| IBIS file p1022_ibis_feb24.ibs generated by Viper version: 2010.02.15
[IBIS Ver]   3.2
[Comment Char]   |_char
[File Name]   p1022_ibis_mar2.ibs
[File Rev]   rev1.0
[Date]   Thu Feb 25 16:07:44 2010
[Source]   Generated using: Viper
[Notes]   updated RLC data
[Disclaimer] IMPORTANT NOTICE
  This information is provided on an AS IS basis and without warranty.
  IN NO EVENT SHALL Freescale BE LIABLE FOR INCIDENTAL OR CONSEQUENTIAL
  DAMAGES ARISING FROM USE OF THIS INFORMATION. THIS DISCLAIMER OF
  WARRANTY EXTENDS TO THE USER OF THE INFORMATION, AND TO THEIR CUSTOMERS
  OR USERS OF PRODUCTS  AND IS IN LIEU OF ALL WARRANTIES WHETHER EXPRESS,
  IMPLIED, OR STATUTORY, INCLUDING IMPLIED WARRANTIES OF MERCHANTABILITY
  OR FITNESS FOR PARTICULAR PURPOSE.
  Freescale does not represent or warrant that the information furnished
  hereunder is free of infringement of any third party patents,
  copyrights, trade secrets, or other intellectual property rights.
  Freescale does not represent or warrant that the information is free of
  defect, or that it meets any particular standard, requirements or need
  of the user of the infomation or their customers.
  Freescale reserves the right to change the information in this file
  without notice.
[Copyright]   (C) Copyright Freescale 2004 - 2010, All Rights Reserved.
|   P1022
[Component]   P1022
[Manufacturer]   FREESCALE
[Package]
| variable   typ   min   max
R_pkg   0.7016960   0.214305   0.869311
L_pkg   7.73384nH   3.69979nH   11.5388nH
C_pkg   1.99730pF   1.32765pF   2.81449pF
[Pin] signal_name   model_name   R_pin   L_pin   C_pin
A1   VSS   GND   NA   NA   NA
A2   VSS   GND   NA   NA   NA
A3   MDQ39   ddr   0.747982  9.70333nH 2.59253pF
A4   GVDD   POWER   NA   NA   NA
A5   MDM05   ddr   0.717482  9.33185nH 1.99975pF
A6   VSS   GND   NA   NA   NA
A7   MDQ47   ddr   0.729467  9.16668nH 2.03973pF
A8   GVDD   POWER   NA   NA   NA
A9   MDQ54   ddr   0.735149  8.13776nH 1.76304pF
A10   GVDD   POWER   NA   NA   NA
A11   MDM07   ddr   0.694958  8.68017nH 1.68609pF
A12   VSS   GND   NA   NA   NA
A13   MDQ63   ddr   0.685751  8.11112nH 1.93324pF
A14   VSS   GND   NA   NA   NA
A15   LAD10   lvcmos   0.777971  8.37697nH 1.67142pF
A16   LAD04   lvcmos   0.700731  8.2178nH  1.9126pF
A17   LAD01   lvcmos   0.75683   8.57406nH 1.87132pF
A18   LAD26   lvcmos   0.760623  8.65983nH 1.85274pF
A19   LAD23   lvcmos   0.766493  8.93644nH 1.743pF
A20   LAD20   lvcmos   0.766971  8.96903nH 1.89829pF
A21   LAD17   lvcmos   0.702347  8.7987nH  1.5871pF
A22   LCS0_B   lvcmos   0.722144  8.74151nH 2.06773pF
A23   VSS   GND   NA   NA   NA
A24   LCLK0   lvcmos   0.808004  9.97666nH 2.20396pF
A25   LCLK1   lvcmos   0.748103  9.5762nH  2.27038pF
A26   VSS   GND   NA   NA   NA
A27   TEMP_CATHODE   POWER   0.751033  9.87414nH 2.26105pF
A28   VSS   GND   NA   NA   NA
A29   VSS   GND   NA   NA   NA
B1   GVDD   POWER   NA   NA   NA
B2   MDQ38   ddr   0.809458  9.97646nH 2.37608pF
B3   VSS   GND   NA   NA   NA
B4   MDQ35   ddr   0.675651  9.29962nH 2.53862pF
B5   MDQ41   ddr   0.754296  9.20264nH 1.96462pF
B6   MDQS05   ddr   0.748763  9.62507nH 2.47055pF
B7   MDQ46   ddr   0.762222  8.92197nH 2.02782pF
B8   MDQ43   ddr   0.708598  8.50501nH 2.08974pF
B9   VSS   GND   NA   NA   NA
B10   MDQ56   ddr   0.741395  8.31025nH 1.94339pF
B11   MDQ57   ddr   0.739117  8.28462nH 1.86747pF
B12   MDQS07   ddr   0.684389  8.73644nH 2.31pF
B13   MDQ62   ddr   0.727662  7.77585nH 1.85543pF
B14   MDQ59   ddr   0.732429  8.00584nH 1.99911pF
B15   LAD11   lvcmos   0.692875  7.49306nH 1.85047pF
B16   LAD05   lvcmos   0.740501  7.94284nH 1.94522pF
B17   LAD02   lvcmos   0.657515  7.76898nH 1.91602pF
B18   VSS   GND   NA   NA   NA
B19   LAD24   lvcmos   0.745003  8.28546nH 1.80061pF
B20   BVDD   POWER   NA   NA   NA
B21   LAD16   lvcmos   0.75217   8.53668nH 1.54649pF
B22   VSS   GND   NA   NA   NA
B23   LWE1_B   lvcmos   0.768453  8.82719nH 1.99814pF
B24   LGPL3   lvcmos   0.720038  8.68977nH 2.09379pF
B25   BVDD   POWER   NA   NA   NA
B26   TEMP_ANODE   POWER   0.800236  9.45775nH 2.23395pF
B27   SPI_CS0_B   lvcmos   0.77681   9.69603nH 2.32325pF
B28   SPI_CS1_B   lvcmos   0.6984   9.31032nH 2.73683pF
B29   VSS   GND   NA   NA   NA
C1   MDQS_B04   ddr   0.792078  9.83271nH 2.57031pF
C2   MDQS04   ddr   0.705702  9.28383nH 2.67801pF
C3   MDM04   ddr   0.71794   9.26539nH 2.42861pF
C4   MDQ34   ddr   0.656881  8.4244nH  2.48774pF
C5   MDQ40   ddr   0.707344  8.62866nH 2.31281pF
C6   MDQS_B05   ddr   0.674196  9.08304nH 2.48388pF
C7   GVDD   POWER   NA   NA   NA
C8   MDQ42   ddr   0.728676  7.7836nH  2.00625pF
C9   MDQS06   ddr   0.653727  7.64321nH 2.03409pF
C10   MDQ60   ddr   0.674331  7.73856nH 2.07298pF
C11   MDQ61   ddr   0.654937  7.13965nH 1.98477pF
C12   MDQS_B07   ddr   0.750121  9.30784nH 2.09011pF
C13   VSS   GND   NA   NA   NA
C14   MDQ58   ddr   0.663714  7.96634nH 1.72058pF
C15   BVDD   POWER   NA   NA   NA
C16   LAD06   lvcmos   0.656701  7.05135nH 1.93021pF
C17   LAD03   lvcmos   0.719406  7.36586nH 1.95061pF
C18   LDP1   lvcmos   0.724029  7.50077nH 1.87876pF
C19   LAD22   lvcmos   0.661298  7.35622nH 1.83935pF
C20   LAD19   lvcmos   0.730113  7.78479nH 1.7538pF
C21   LCS2_B   lvcmos   0.739806  7.92256nH 1.93931pF
C22   LGPL0   lvcmos   0.745588  8.03202nH 2.076pF
C23   LALE   lvcmos   0.750517  8.2294nH  2.09312pF
C24   LGPL4   lvcmos   0.765139  8.58843nH 2.06771pF
C25   SPI_MOSI   lvcmos   0.705009  8.35195nH 2.26877pF
C26   VSS   GND   NA   NA   NA
C27   SPI_CS2_B   lvcmos   0.734144  9.07613nH 2.2447pF
C28   SDHC_DAT1   lvcmos   0.696295  9.23289nH 2.50112pF
C29   SDHC_CLK   lvcmos   0.831498  10.5218nH 2.28529pF
D1   GVDD   POWER   NA   NA   NA
D2   MDQ37   ddr   0.76027   9.50741nH 2.12906pF
D3   MDQ33   ddr   0.807158  9.50311nH 2.13208pF
D4   MDQ44   ddr   0.627315  7.98496nH 2.36865pF
D5   VSS   GND   NA   NA   NA
D6   MDQ45   ddr   0.620035  7.41491nH 2.27755pF
D7   MDQ48   ddr   0.712654  7.33209nH 2.20401pF
D8   MDQ49   ddr   0.71175   7.38798nH 1.96456pF
D9   MDQS_B06   ddr   0.719441  7.97825nH 2.07488pF
D10   GVDD   POWER   NA   NA   NA
D11   MDQ51   ddr   0.731452  7.99976nH 1.93683pF
D12   GVDD   POWER   NA   NA   NA
D13   LAD14   lvcmos   0.687323  6.47207nH 1.51203pF
D14   LAD13   lvcmos   0.643595  6.56045nH 1.6414pF
D15   LAD12   lvcmos   0.710721  6.70823nH 1.78542pF
D16   LAD07   lvcmos   0.69999   6.92713nH 1.83412pF
D17   VSS   GND   NA   NA   NA
D18   LAD27   lvcmos   0.644075  6.59265nH 1.76486pF
D19   BVDD   POWER   NA   NA   NA
D20   LAD18   lvcmos   0.71132   7.2312nH  1.79978pF
D21   VSS   GND   NA   NA   NA
D22   LBCTL   lvcmos   0.662836  6.99163nH 2.16362pF
D23   BVDD   POWER   NA   NA   NA
D24   LGPL5   lvcmos   0.685726  7.65156nH 2.17734pF
D25   SPI_CLK   lvcmos   0.667534  7.73941nH 2.15435pF
D26   SDHC_DAT0   lvcmos   0.722686  8.33496nH 2.81449pF
D27   SDHC_DAT2   lvcmos   0.769674  9.19593nH 2.36132pF
D28   UART_SIN0   lvcmos   0.818963  9.51209nH 2.34724pF
D29   VSS   GND   NA   NA   NA
E1   MODT01   ddr   0.768945  9.58951nH 2.06186pF
E2   MODT03   ddr   0.745012  9.04779nH 2.23177pF
E3   VSS   GND   NA   NA   NA
E4   MDQ36   ddr   0.71465   8.3374nH  2.12026pF
E5   MDQ32   ddr   0.723452  8.04595nH 2.22862pF
E6   GVDD   POWER   NA   NA   NA
E7   MDQ52   ddr   0.651886  7.21957nH 1.96438pF
E8   GVDD   POWER   NA   NA   NA
E9   VSS   GND   NA   NA   NA
E10   MDQ55   ddr   0.694918  6.93545nH 1.8336pF
E11   VSS   GND   NA   NA   NA
E12   MDIC00   ddr   0.671948  5.99856nH 1.66456pF
E13   LAD15   lvcmos   0.631894  6.71174nH 1.63833pF
E14   VSS   GND   NA   NA   NA
E15   BVDD   POWER   NA   NA   NA
E16   LAD09   lvcmos   0.619147  5.85899nH 1.8411pF
E17   LAD08   lvcmos   0.623017  5.91538nH 1.856pF
E18   LAD00   lvcmos   0.622408  6.07334nH 1.7523pF
E19   LAD21   lvcmos   0.626555  6.12834nH 1.9256pF
E20   LCS1_B   lvcmos   0.635442  6.17821nH 1.82914pF
E21   LWE0_B   lvcmos   0.638292  6.39312nH 2.00511pF
E22   LGPL2   lvcmos   0.711723  7.01223nH 2.1374pF
E23   DIU_DE   lvcmos   0.718933  7.195nH   2.22906pF
E24   VSS   GND   NA   NA   NA
E25   SPI_CS3_B   lvcmos   0.593703  6.90482nH 2.23741pF
E26   SDHC_DAT3   lvcmos   0.663694  7.64798nH 2.35593pF
E27   OVDD   POWER   NA   NA   NA
E28   UART_SIN1   lvcmos   0.814474  9.39955nH 2.28045pF
E29   SSI_TXD   lvcmos   0.773615  9.5324nH  2.30058pF
F1   MODT00   ddr   0.767477  9.43676nH 2.13559pF
F2   MODT02   ddr   0.81492   9.35608nH 2.1323pF
F3   MA13   ddr   0.784095  8.73301nH 2.18083pF
F4   VSS   GND   NA   NA   NA
F5   MCS_B01   ddr   0.749609  7.70032nH 2.17327pF
F6   MCS_B03   ddr   0.73552   7.35365nH 2.19972pF
F7   VSS   GND   NA   NA   NA
F8   MDQ53   ddr   0.643059  6.74904nH 2.00573pF
F9   GVDD   POWER   NA   NA   NA
F10   MDM06   ddr   0.636797  6.68012nH 2.05382pF
F11   MDQ50   ddr   0.632859  6.51846nH 2.07728pF
F12   MDIC01   ddr   0.593766  6.03687nH 1.60187pF
F13   VSS   GND   NA   NA   NA
F14   SENSEVDD   POWER   0.628311  5.49999nH 1.65526pF
F15   SENSEVSS   GND   NA   NA   NA
F16   BVDD   POWER   NA   NA   NA
F17   LDP0   lvcmos   0.607637  5.50127nH 1.79259pF
F18   LAD25   lvcmos   0.594032  5.39975nH 1.72445pF
F19   LCS3_B   lvcmos   0.62234   5.84429nH 1.83376pF
F20   BVDD   POWER   NA   NA   NA
F21   LGPL1   lvcmos   0.62597   5.69382nH 1.58857pF
F22   BVDD   POWER   NA   NA   NA
F23   SPI_MISO   lvcmos   0.694828  6.68908nH 1.77993pF
F24   SDHC_CMD   lvcmos   0.581608  6.4253nH  2.77594pF
F25   SDHC_WP   lvcmos   0.736041  7.52883nH 2.1004pF
F26   SSI_TFS   lvcmos   0.776554  8.45125nH 1.93089pF
F27   UART_RTS0_B   lvcmos   0.791654  8.73106nH 2.23647pF
F28   UART_SOUT0   lvcmos   0.735462  8.53016nH 2.17307pF
F29   OVDD   POWER   NA   NA   NA
G1   MWE_B   ddr   0.81798   9.63755nH 2.09559pF
G2   MCS_B00   ddr   0.73876   8.49107nH 2.12548pF
G3   GVDD   POWER   NA   NA   NA
G4   MCS_B02   ddr   0.675974  7.31698nH 2.09895pF
G5   VSS   GND   NA   NA   NA
G6   MCAS_B   ddr   0.670224  6.89342nH 2.23097pF
G9   AVDD_CORE0   POWER   0.310257  5.00716nH 2.08432pF
G10   VSS   GND   NA   NA   NA
G20   AVDD_CORE1   POWER   0.235846  3.9426nH  1.77074pF
G21   VSS   GND   NA   NA   NA
G24   SDHC_CD   lvcmos   0.615851  5.79493nH 1.8637pF
G25   OVDD   POWER   NA   NA   NA
G26   SSI_TCK   lvcmos   0.67726   7.08006nH 1.88322pF
G27   VSS   GND   NA   NA   NA
G28   IIC1_SCL   lvcmos   0.731176  8.33606nH 1.99554pF
G29   CKSTP_IN1_B   lvcmos   0.810997  9.63909nH 1.96353pF
H1   VSS   GND   NA   NA   NA
H2   MCK_B00   ddr   0.68165   7.52908nH 2.11178pF
H3   MCK00   ddr   0.750375  8.08883nH 2.14795pF
H4   VSS   GND   NA   NA   NA
H5   MBA00   ddr   0.742889  7.21161nH 1.88577pF
H6   MRAS_B   ddr   0.652761  6.3406nH  2.02834pF
H24   UART_SOUT1   lvcmos   0.650936  6.02915nH 2.17556pF
H25   CKSTP_IN0_B   lvcmos   0.67136   6.76601nH 2.04482pF
H26   UART_RTS1_B   lvcmos   0.756241  7.7748nH  1.95949pF
H27   CKSTP_OUT0_B   lvcmos   0.706241  8.02652nH 2.07119pF
H28   UDE1_B   lvcmos   0.712269  8.21792nH 2.17731pF
H29   VSS   GND   NA   NA   NA
J1   MA00   ddr   0.796246  9.22816nH 1.84503pF
J2   VSS   GND   NA   NA   NA
J3   GVDD   POWER   NA   NA   NA
J4   MA10   ddr   0.686989  7.12046nH 1.84029pF
J5   MBA01   ddr   0.734781  6.97896nH 1.77277pF
J6   GVDD   POWER   NA   NA   NA
J7   MVREF   POWER   0.267911  3.89422nH 2.45211pF
J23   UART_CTS1_B   lvcmos   0.629162  5.35462nH 2.03577pF
J24   IIC1_SDA   lvcmos   0.639074  5.71514nH 1.9761pF
J25   OVDD   POWER   NA   NA   NA
J26   IRQ10   lvcmos   0.67645   7.06237nH 2.08085pF
J27   IRQ11   lvcmos   0.754726  8.10729nH 2.08486pF
J28   IRQ_OUT_B   lvcmos   0.758499  8.45336nH 1.95538pF
J29   SRESET_B   lvcmos   0.869311  11.5388nH 2.11591pF
K1   GVDD   POWER   NA   NA   NA
K2   MCK02   ddr   0.665769  7.15095nH 2.13736pF
K3   MCK_B02   ddr   0.726796  7.62398nH 2.00158pF
K4   GVDD   POWER   NA   NA   NA
K5   MA01   ddr   0.708382  6.56449nH 1.78235pF
K6   VSS   GND   NA   NA   NA
K7   VSS   GND   NA   NA   NA
K10   VDD   POWER   NA   NA   NA
K11   VDD   POWER   NA   NA   NA
K12   VDD   POWER   NA   NA   NA
K13   VDD   POWER   NA   NA   NA
K14   VDD   POWER   NA   NA   NA
K15   VDD   POWER   NA   NA   NA
K16   VDD   POWER   NA   NA   NA
K17   VDD   POWER   NA   NA   NA
K18   VDD   POWER   NA   NA   NA
K19   VDD   POWER   NA   NA   NA
K20   VDD   POWER   NA   NA   NA
K23   VSS   GND   NA   NA   NA
K24   UART_CTS0_B   lvcmos   0.693565  5.94257nH 1.83568pF
K25   MCP1_B   lvcmos   0.699642  6.50366nH 2.07126pF
K26   MCP0_B   lvcmos   0.66247   6.85144nH 2.1763pF
K27   IRQ06   lvcmos   0.681091  7.56841nH 2.1623pF
K28   IRQ08   lvcmos   0.76863   8.68056nH 2.1677pF
K29   OVDD   POWER   NA   NA   NA
L1   MCK_B03   ddr   0.734922  8.03983nH 2.05312pF
L2   MCK03   ddr   0.67263   7.55603nH 2.02095pF
L3   VSS   GND   NA   NA   NA
L4   MA03   ddr   0.727973  7.28074nH 1.7884pF
L5   GVDD   POWER   NA   NA   NA
L6   MA02   ddr   0.629357  5.53765nH 1.6768pF
L10   VDD   POWER   NA   NA   NA
L11   VSS   GND   NA   NA   NA
L12   VSS   GND   NA   NA   NA
L13   VSS   GND   NA   NA   NA
L14   VSS   GND   NA   NA   NA
L15   VSS   GND   NA   NA   NA
L16   VSS   GND   NA   NA   NA
L17   VSS   GND   NA   NA   NA
L18   VSS   GND   NA   NA   NA
L19   VSS   GND   NA   NA   NA
L20   VDD   POWER   NA   NA   NA
L24   CKSTP_OUT1_B   lvcmos   0.689227  6.02751nH 1.83644pF
L25   TRIG_IN   lvcmos   0.69154   6.35757nH 1.71564pF
L26   VSS   GND   NA   NA   NA
L27   READY_P1   lvcmos   0.727793  7.67494nH 1.94516pF
L28   IRQ09   lvcmos   0.669829  7.35824nH 2.016pF
L29   TRST_B   lvcmos   0.75249   8.62062nH 1.87616pF
M1   VSS   GND   NA   NA   NA
M2   MA06   ddr   0.747102  7.96217nH 2.03621pF
M3   MA08   ddr   0.668586  6.99082nH 1.96255pF
M4   VSS   GND   NA   NA   NA
M5   MA05   ddr   0.676039  5.77571nH 1.60285pF
M6   MA04   ddr   0.616647  5.3732nH  1.62193pF
M10   VDD   POWER   NA   NA   NA
M11   VSS   GND   NA   NA   NA
M12   VSS   GND   NA   NA   NA
M13   VSS   GND   NA   NA   NA
M14   VSS   GND   NA   NA   NA
M15   VSS   GND   NA   NA   NA
M16   VSS   GND   NA   NA   NA
M17   VSS   GND   NA   NA   NA
M18   VSS   GND   NA   NA   NA
M19   VSS   GND   NA   NA   NA
M20   VDD   POWER   NA   NA   NA
M24   UDE0_B   lvcmos   0.604684  5.30535nH 1.82263pF
M25   TRIG_OUT   lvcmos   0.605211  5.52842nH 1.69668pF
M26   TMS   lvcmos   0.680323  6.47272nH 1.71661pF
M27   TEST_SEL_B   lvcmos   0.641802  6.5438nH  2.01703pF
M28   TDO   lvcmos   0.661586  7.48518nH 1.77687pF
M29   CLK_OUT   lvcmos   0.74508   9.50959nH 2.26363pF
N1   MA07   ddr   0.760278  8.53997nH 1.82525pF
N2   GVDD   POWER   NA   NA   NA
N3   MCK04   ddr   0.62391   6.12413nH 1.8762pF
N4   MCK_B04   ddr   0.689124  6.60337nH 1.94903pF
N5   MA11   ddr   0.629666  5.97326nH 1.7484pF
N6   GVDD   POWER   NA   NA   NA
N10   VDD   POWER   NA   NA   NA
N11   VSS   GND   NA   NA   NA
N12   VSS   GND   NA   NA   NA
N13   VSS   GND   NA   NA   NA
N14   VSS   GND   NA   NA   NA
N15   VSS   GND   NA   NA   NA
N16   VSS   GND   NA   NA   NA
N17   VSS   GND   NA   NA   NA
N18   VSS   GND   NA   NA   NA
N19   VSS   GND   NA   NA   NA
N20   VDD   POWER   NA   NA   NA
N24   O2VDD   POWER   NA   NA   NA
N25   IRQ07   lvcmos   0.706639  7.122nH   1.78275pF
N26   TCK   lvcmos   0.632794  6.45982nH 1.6978pF
N27   OVDD   POWER   NA   NA   NA
N28   TDI   lvcmos   0.669808  7.83522nH 1.92322pF
N29   VSS   GND   NA   NA   NA
P1   MA09   ddr   0.761782  8.66565nH 1.91017pF
P2   MA12   ddr   0.734634  7.84455nH 1.77566pF
P3   GVDD   POWER   NA   NA   NA
P4   MA14   ddr   0.640481  6.35886nH 1.88735pF
P5   VSS   GND   NA   NA   NA
P6   MA15   ddr   0.600726  5.18608nH 1.6909pF
P10   VDDC   POWER   NA   NA   NA
P11   VSS   GND   NA   NA   NA
P12   VSS   GND   NA   NA   NA
P13   VSS   GND   NA   NA   NA
P14   VSS   GND   NA   NA   NA
P15   VSS   GND   NA   NA   NA
P16   VSS   GND   NA   NA   NA
P17   VSS   GND   NA   NA   NA
P18   VSS   GND   NA   NA   NA
P19   VSS   GND   NA   NA   NA
P20   VDD   POWER   NA   NA   NA
P24   AVDD_PLAT   POWER   0.225725  3.91717nH 1.70343pF
P25   BVDD_VSEL1   lvcmos   0.583695  5.28241nH 1.66388pF
P26   SCAN_MODE_B   lvcmos   0.723151  7.58863nH 2.37353pF
P27   HRESET_B   lvcmos   0.626681  6.547nH   1.76201pF
P28   HRESET_REQ_B   lvcmos   0.724556  7.83466nH 1.78084pF
P29   SYS_CLK_IN   lvcmos   0.744299  8.45424nH 1.65183pF
R1   MECC03   ddr   0.696247  8.27557nH 1.97882pF
R2   MECC07   ddr   0.73996   8.13322nH 1.94202pF
R3   MCK01   ddr   0.621499  6.22548nH 1.78015pF
R4   MCK_B01   ddr   0.686242  6.72345nH 1.84929pF
R5   GVDD   POWER   NA   NA   NA
R6   MBA02   ddr   0.587662  4.86479nH 1.66315pF
R10   VDDC   POWER   NA   NA   NA
R11   VSS   GND   NA   NA   NA
R12   VSS   GND   NA   NA   NA
R13   VSS   GND   NA   NA   NA
R14   VSS   GND   NA   NA   NA
R15   VSS   GND   NA   NA   NA
R16   VSS   GND   NA   NA   NA
R17   VSS   GND   NA   NA   NA
R18   VSS   GND   NA   NA   NA
R19   VSS   GND   NA   NA   NA
R20   VDD   POWER   NA   NA   NA
R24   POWER_OK   lvcmos   0.586072  5.21871nH 1.74996pF
R25   VSS   GND   NA   NA   NA
R26   BVDD_VSEL0   lvcmos   0.668531  6.22835nH 1.78343pF
R27   LVDD_VSEL   lvcmos   0.639598  6.84039nH 1.83973pF
R28   SENSEVDDC   POWER   0.667936  7.68638nH 1.76873pF
R29   O2VDD   POWER   NA   NA   NA
T1   MECC02   ddr   0.74095   8.15796nH 1.92604pF
T2   MECC06   ddr   0.67143   7.48077nH 1.88371pF
T3   VSS   GND   NA   NA   NA
T4   MCK05   ddr   0.671192  6.22963nH 1.85988pF
T5   MCK_B05   ddr   0.604507  5.63884nH 1.97876pF
T6   VSS   GND   NA   NA   NA
T10   VDD   POWER   NA   NA   NA
T11   VSS   GND   NA   NA   NA
T12   VSS   GND   NA   NA   NA
T13   VSS   GND   NA   NA   NA
T14   VSS   GND   NA   NA   NA
T15   VSS   GND   NA   NA   NA
T16   VSS   GND   NA   NA   NA
T17   VSS   GND   NA   NA   NA
T18   VSS   GND   NA   NA   NA
T19   VSS   GND   NA   NA   NA
T20   VDD1C   POWER   NA   NA   NA
T24   IRQ05   lvcmos   0.589086  5.2944nH  1.95022pF
T25   ASLEEP   lvcmos   0.667301  6.10241nH 1.63205pF
T26   IRQ00   lvcmos   0.687158  6.76086nH 1.74101pF
T27   O2VDD   POWER   NA   NA   NA
T28   IRQ04   lvcmos   0.726744  8.01525nH 1.73347pF
T29   RTC_CLK   lvcmos   0.69783   8.57303nH 1.96035pF
U1   VSS   GND   NA   NA   NA
U2   MDQS08   ddr   0.716988  7.89065nH 1.98034pF
U3   MDQS_B08   ddr   0.652329  7.35067nH 2.09729pF
U4   MCKE01   ddr   0.705471  6.98965nH 1.98496pF
U5   GVDD   POWER   NA   NA   NA
U6   MCKE00   ddr   0.592512  5.08767nH 1.81435pF
U10   VDD   POWER   NA   NA   NA
U11   VSS   GND   NA   NA   NA
U12   VSS   GND   NA   NA   NA
U13   VSS   GND   NA   NA   NA
U14   VSS   GND   NA   NA   NA
U15   VSS   GND   NA   NA   NA
U16   VSS   GND   NA   NA   NA
U17   VSS   GND   NA   NA   NA
U18   VSS   GND   NA   NA   NA
U19   VSS   GND   NA   NA   NA
U20   VDD1C   POWER   NA   NA   NA
U24   IRQ03   lvcmos   0.601269  5.57921nH 1.84659pF
U25   VSS   GND   NA   NA   NA
U26   USB1_NXT   lvcmos   0.629338  6.45057nH 1.69032pF
U27   POWER_EN   lvcmos   0.644821  7.00555nH 1.74565pF
U28   IRQ01   lvcmos   0.729463  8.04877nH 1.86148pF
U29   IRQ02   lvcmos   0.752273  8.79128nH 1.80881pF
V1   MDM08   ddr   0.746958  8.29642nH 1.83805pF
V2   MECC01   ddr   0.668827  7.31868nH 1.90491pF
V3   VSS   GND   NA   NA   NA
V4   MCKE02   ddr   0.711189  7.17234nH 1.94967pF
V5   VSS   GND   NA   NA   NA
V6   MCKE03   ddr   0.605909  5.48656nH 1.80924pF
V10   VDD   POWER   NA   NA   NA
V11   VSS   GND   NA   NA   NA
V12   VSS   GND   NA   NA   NA
V13   VSS   GND   NA   NA   NA
V14   VSS   GND   NA   NA   NA
V15   VSS   GND   NA   NA   NA
V16   VSS   GND   NA   NA   NA
V17   VSS   GND   NA   NA   NA
V18   VSS   GND   NA   NA   NA
V19   VSS   GND   NA   NA   NA
V20   VDD   POWER   NA   NA   NA
V24   USB1_D3   lvcmos   0.607322  5.71096nH 1.75879pF
V25   USB1_D1   lvcmos   0.65881   5.76643nH 1.66699pF
V26   USB1_D0   lvcmos   0.618288  6.01963nH 1.89407pF
V27   L2VDD   POWER   NA   NA   NA
V28   USB1_DIR   lvcmos   0.715894  7.56709nH 1.98495pF
V29   USB1_STP   lvcmos   0.752319  8.69895nH 1.6905pF
W1   GVDD   POWER   NA   NA   NA
W2   MECC05   ddr   0.731698  7.85348nH 1.90405pF
W3   MECC00   ddr   0.65613   6.92897nH 1.99099pF
W4   VSS   GND   NA   NA   NA
W5   MDQ27   ddr   0.702912  6.60364nH 1.93405pF
W6   VSS   GND   NA   NA   NA
W10   VDD   POWER   NA   NA   NA
W11   VSS   GND   NA   NA   NA
W12   VSS   GND   NA   NA   NA
W16   VSS   GND   NA   NA   NA
W18   VSS   GND   NA   NA   NA
W19   VSS   GND   NA   NA   NA
W20   VDD   POWER   NA   NA   NA
W24   USB1_D5   lvcmos   0.620582  6.10759nH 1.88772pF
W25   VSS   GND   NA   NA   NA
W26   USB1_D4   lvcmos   0.711238  7.34956nH 1.81292pF
W27   USB1_CLK   lvcmos   0.673707  7.77621nH 1.87247pF
W28   USB1_D2   lvcmos   0.74607   8.38541nH 1.79201pF
W29   VSS   GND   NA   NA   NA
Y1   MECC04   ddr   0.744797  8.23151nH 1.9271pF
Y2   MDQ19   ddr   0.703654  8.40512nH 2.13386pF
Y3   VSS   GND   NA   NA   NA
Y4   MDQ26   ddr   0.645595  6.29946nH 1.83215pF
Y5   MDQ31   ddr   0.716708  6.94691nH 1.80488pF
Y6   GVDD   POWER   NA   NA   NA
Y7   GVDD   POWER   NA   NA   NA
Y10   AVDD_DDR   POWER   0.214305  3.69979nH 1.95615pF
Y11   VDD   POWER   NA   NA   NA
Y12   VDD   POWER   NA   NA   NA
Y16   VDD   POWER   NA   NA   NA
Y18   VDD   POWER   NA   NA   NA
Y19   VDD   POWER   NA   NA   NA
Y20   VDD   POWER   NA   NA   NA
Y23   VSS   GND   NA   NA   NA
Y24   USB1_D7   lvcmos   0.617006  6.02818nH 1.96398pF
Y25   USB1_D6   lvcmos   0.697804  6.9541nH  1.80869pF
Y26   TSEC1_RXD2   lvcmos   0.715351  7.38259nH 1.75853pF
Y27   L2VDD   POWER   NA   NA   NA
Y28   TSEC1_RXD1   lvcmos   0.688816  7.99755nH 1.91339pF
Y29   TSEC1_GTX_CLK125   lvcmos   0.771088  9.03453nH 1.87871pF
AA1   MDQ18   ddr   0.795809  9.69339nH 2.17107pF
AA2   MDQ23   ddr   0.709076  8.49571nH 2.17933pF
AA3   MDQ22   ddr   0.771421  8.9429nH  2.1567pF
AA4   GVDD   POWER   NA   NA   NA
AA5   MDQ30   ddr   0.6549   6.57618nH 1.87999pF
AA6   MDM03   ddr   0.66511   6.7596nH  2.0776pF
AA7   VSS   GND   NA   NA   NA
AA23  TSEC1_RXD3   lvcmos   0.689364  6.28487nH 1.98785pF
AA24  TSEC1_RX_DV   lvcmos   0.722191  7.43464nH 1.96713pF
AA25  L2VDD   POWER   NA   NA   NA
AA26  TSEC1_RXD0   lvcmos   0.662609  7.05028nH 1.86096pF
AA27  TSEC1_TXD3   lvcmos   0.752433  8.17827nH 2.01611pF
AA28  TSEC1_TX_EN   lvcmos   0.719164  8.93363nH 2.05205pF
AA29  VSS   GND   NA   NA   NA
AB1   VSS   GND   NA   NA   NA
AB2   MDQS02   ddr   0.751456  8.86427nH 2.41421pF
AB3   MDQS_B02   ddr   0.687495  8.3718nH  2.47445pF
AB4   MDQS_B03   ddr   0.646093  6.5114nH  2.21966pF
AB5   MDQS03   ddr   0.708597  7.03821nH 2.25397pF
AB6   GVDD   POWER   NA   NA   NA
AB24  TSEC2_RX_CLK   lvcmos   0.69745   6.16275nH 1.7061pF
AB25  TSEC1_TXD2   lvcmos   0.730216  7.19852nH 2.02132pF
AB26  VSS   GND   NA   NA   NA
AB27  TSEC1_TXD0   lvcmos   0.763196  8.31969nH 1.92929pF
AB28  TSEC1_TXD1   lvcmos   0.710356  8.2521nH  2.02809pF
AB29  TSEC1_RX_CLK   lvcmos   0.724709  8.99529nH 1.95072pF
AC1   MDM02   ddr   0.720921  8.90853nH 2.00523pF
AC2   MDQ17   ddr   0.791928  9.39064nH 2.15356pF
AC3   MDQ21   ddr   0.777352  8.80939nH 2.26867pF
AC4   VSS   GND   NA   NA   NA
AC5   MDQ25   ddr   0.738948  7.43405nH 1.92245pF
AC6   MDQ29   ddr   0.736137  7.39419nH 2.18276pF
AC20  SD_IMP_CAL_TX2   tx_pzctl   0.698084  5.35753nH 1.85591pF
AC21  X2VSS   GND   NA   NA   NA
AC24  TSEC2_TXD0   lvcmos   0.62913   6.59453nH 2.02328pF
AC25  LVDD   POWER   NA   NA   NA
AC26  TSEC2_GTX_CLK   lvcmos   0.756982  7.92708nH 2.05207pF
AC27  TSEC2_RXD3   lvcmos   0.75544   8.04661nH 2.17475pF
AC28  TSEC2_RX_DV   lvcmos   0.709701  8.08989nH 2.19683pF
AC29  VSS   GND   NA   NA   NA
AD1   MDQ16   ddr   0.747121  9.47092nH 2.23892pF
AD2   MDQ20   ddr   0.73457   8.97058nH 2.35503pF
AD3   GVDD   POWER   NA   NA   NA
AD4   MDQ28   ddr   0.757823  8.00645nH 1.98016pF
AD5   MDQ24   ddr   0.691876  7.46687nH 2.01299pF
AD6   VSS   GND   NA   NA   NA
AD7   DDRCLK   lvcmos   0.725731  7.80904nH 1.81614pF
AD8   XVSS   GND   NA   NA   NA
AD9   SD_TXA_P   lynx_tx   0.767153  7.41281nH 1.57434pF
AD10  XVDD   POWER   NA   NA   NA
AD11  SDAVDD   POWER   0.665957  7.35563nH 1.39528pF
AD12  SDAVSS   GND   NA   NA   NA
AD13  SD_PLL_TPA   opdalg_out   0.661314  6.02375nH 1.54654pF
AD14  XVDD   POWER   NA   NA   NA
AD15  SD_TXF_P   lynx_tx   0.723625  6.18732nH 1.32765pF
AD16  XVSS   GND   NA   NA   NA
AD17  X2VSS   GND   NA   NA   NA
AD18  SD_PLL_TPD2   pouv_out   0.672646  5.57979nH 1.66844pF
AD19  SDAVDD2   POWER   0.638341  6.25359nH 1.59881pF
AD20  X2VSS   GND   NA   NA   NA
AD21  SD_TXE_N2   lynx_tx   0.734851  6.65032nH 1.7116pF
AD22  X2VDD   POWER   NA   NA   NA
AD23  VSS   GND   NA   NA   NA
AD24  TSEC_1588_CLK_OUT   lvcmos   0.66378   6.98275nH 2.72173pF
AD25  TSEC2_TXD1   lvcmos   0.746153  8.30497nH 2.80784pF
AD26  FA_VDD   POWER   0.761131  8.05443nH 2.19663pF
AD27  TSEC2_RXD2   lvcmos   0.715598  8.22195nH 2.13812pF
AD28  POVDD   POWER   0.730029  8.63467nH 1.9705pF
AD29  TSEC1_GTX_CLK   lvcmos   0.749816  9.2186nH  2.21955pF
AE1   VSS   GND   NA   NA   NA
AE2   MDQ11   ddr   0.752689  9.44986nH 2.10991pF
AE3   MDQ10   ddr   0.79641   9.30975nH 2.071pF
AE4   VSS   GND   NA   NA   NA
AE5   MDQ15   ddr   0.622086  7.14341nH 2.26945pF
AE6   MDQ14   ddr   0.675537  9.03836nH 2.40484pF
AE7   VSS   GND   NA   NA   NA
AE8   XVDD   POWER   NA   NA   NA
AE9   SD_TXA_N   lynx_tx   0.776672  7.05759nH 1.73301pF
AE10  SD_TXB_P   lynx_tx   0.694223  7.03079nH 1.77516pF
AE11  XVSS   GND   NA   NA   NA
AE12  SD_PLL_TPD   pouv_out   0.743327  6.15765nH 1.67568pF
AE13  XVSS   GND   NA   NA   NA
AE14  SD_TXE_P   lynx_tx   0.663139  7.05245nH 1.6831pF
AE15  SD_TXF_N   lynx_tx   0.727544  6.01318nH 1.49367pF
AE16  XVDD   POWER   NA   NA   NA
AE17  SD_TXA_P2   lynx_tx   0.736953  6.83502nH 1.44397pF
AE18  X2VDD   POWER   NA   NA   NA
AE19  SDAVSS2   GND   NA   NA   NA
AE20  X2VSS   GND   NA   NA   NA
AE21  SD_TXE_P2   lynx_tx   0.735237  6.65822nH 1.74802pF
AE22  X2VDD   POWER   NA   NA   NA
AE23  VSS   GND   NA   NA   NA
AE24  TSEC_1588_PULSE_OUT1 lvcmos   0.583265  6.98743nH 2.71577pF
AE25  LVDD   POWER   NA   NA   NA
AE26  TSEC2_TX_EN   lvcmos   0.781846  8.8613nH  2.0133pF
AE27  VSS   GND   NA   NA   NA
AE28  TSEC2_RXD1   lvcmos   0.816418  9.65856nH 2.25875pF
AE29  LVDD   POWER   NA   NA   NA
AF1   MDQS01   ddr   0.74139   10.8726nH 2.72838pF
AF2   GVDD   POWER   NA   NA   NA
AF3   MDM01   ddr   0.791041  9.38409nH 2.37806pF
AF4   MDQ08   ddr   0.740629  8.79748nH 2.27745pF
AF5   MDQ12   ddr   0.716996  8.35449nH 2.38214pF
AF6   GVDD   POWER   NA   NA   NA
AF7   VSS   GND   NA   NA   NA
AF8   XVSS   GND   NA   NA   NA
AF9   XVSS   GND   NA   NA   NA
AF10  SD_TXB_N   lynx_tx   0.698896  6.93622nH 1.80151pF
AF11  XVDD   POWER   NA   NA   NA
AF12  SD_REF_CLK_B   ptrmr100_cm   0.704775  7.61118nH 1.70107pF
AF13  XVDD   POWER   NA   NA   NA
AF14  SD_TXE_N   lynx_tx   0.659113  6.50531nH 1.65965pF
AF15  XVSS   GND   NA   NA   NA
AF16  SD_IMP_CAL_TX   tx_pzctl   0.726209  6.62944nH 1.79653pF
AF17  SD_TXA_N2   lynx_tx   0.735773  6.79387nH 1.50033pF
AF18  S2VSS   GND   NA   NA   NA
AF19  SD_PLL_TPA2   opdalg_out   0.7577   6.94577nH 1.82348pF
AF20  X2VDD   POWER   NA   NA   NA
AF21  S2VSS   GND   NA   NA   NA
AF22  X2VSS   GND   NA   NA   NA
AF24  VSS   GND   NA   NA   NA
AF25  VSS   GND   NA   NA   NA
AF26  TSEC_1588_ALARM_OUT1 lvcmos   0.640101  8.1342nH  2.27843pF
AF27  TSEC2_TXD3   lvcmos   0.717311  8.94031nH 2.29889pF
AF28  VSS   GND   NA   NA   NA
AF29  TSEC2_RXD0   lvcmos   0.777582  9.96458nH 2.2087pF
AG1   MDQS_B01   ddr   0.811159  11.4708nH 2.54042pF
AG2   MDQ09   ddr   0.751936  9.77961nH 2.19936pF
AG3   MDQ03   ddr   0.679181  8.92513nH 2.58718pF
AG4   VSS   GND   NA   NA   NA
AG5   MDQS00   ddr   0.703516  9.84203nH 2.74267pF
AG6   MDQ01   ddr   0.687546  8.33583nH 2.25869pF
AG7   VSS   GND   NA   NA   NA
AG8   SD_IMP_CAL_RX   rx_pzctl   0.802968  8.32078nH 1.97143pF
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[Pin Mapping]   pulldown_ref   pullup_ref
A1   VSS   NC
A2   VSS   NC
A3   NC   GVDD
A4   NC   GVDD
A5   NC   GVDD
A6   VSS   NC
A7   NC   GVDD
A8   NC   GVDD
A9   NC   GVDD
A10   NC   GVDD
A11   NC   GVDD
A12   VSS   NC
A13   NC   GVDD
A14   VSS   NC
A15   NC   BVDD
A16   NC   BVDD
A17   NC   BVDD
A18   NC   BVDD
A19   NC   BVDD
A20   NC   BVDD
A21   NC   BVDD
A22   NC   BVDD
A23   VSS   NC
A24   NC   BVDD
A25   NC   BVDD
A26   VSS   NC
A27   NC   BVDD
A28   VSS   NC
A29   VSS   NC
B1   NC   GVDD
B2   NC   GVDD
B3   VSS   NC
B4   NC   GVDD
B5   NC   GVDD
B6   NC   GVDD
B7   NC   GVDD
B8   NC   GVDD
B9   VSS   NC
B10   NC   GVDD
B11   NC   GVDD
B12   NC   GVDD
B13   NC   GVDD
B14   NC   GVDD
B15   NC   BVDD
B16   NC   BVDD
B17   NC   BVDD
B18   VSS   NC
B19   NC   BVDD
B20   NC   BVDD
B21   NC   BVDD
B22   VSS   NC
B23   NC   BVDD
B24   NC   BVDD
B25   NC   BVDD
B26   NC   BVDD
B27   NC   BVDD
B28   NC   BVDD
B29   VSS   NC
C1   NC   GVDD
C2   NC   GVDD
C3   NC   GVDD
C4   NC   GVDD
C5   NC   GVDD
C6   NC   GVDD
C7   NC   GVDD
C8   NC   GVDD
C9   NC   GVDD
C10   NC   GVDD
C11   NC   GVDD
C12   NC   GVDD
C13   VSS   NC
C14   NC   GVDD
C15   NC   BVDD
C16   NC   BVDD
C17   NC   BVDD
C18   NC   BVDD
C19   NC   BVDD
C20   NC   BVDD
C21   NC   BVDD
C22   NC   BVDD
C23   NC   BVDD
C24   NC   BVDD
C25   NC   BVDD
C26   VSS   NC
C27   NC   BVDD
C28   NC   OVDD
C29   NC   OVDD
D1   NC   GVDD
D2   NC   GVDD
D3   NC   GVDD
D4   NC   GVDD
D5   VSS   NC
D6   NC   GVDD
D7   NC   GVDD
D8   NC   GVDD
D9   NC   GVDD
D10   NC   GVDD
D11   NC   GVDD
D12   NC   GVDD
D13   NC   BVDD
D14   NC   BVDD
D15   NC   BVDD
D16   NC   BVDD
D17   VSS   NC
D18   NC   BVDD
D19   NC   BVDD
D20   NC   BVDD
D21   VSS   NC
D22   NC   BVDD
D23   NC   BVDD
D24   NC   BVDD
D25   NC   BVDD
D26   NC   OVDD
D27   NC   OVDD
D28   NC   OVDD
D29   VSS   NC
E1   NC   GVDD
E2   NC   GVDD
E3   VSS   NC
E4   NC   GVDD
E5   NC   GVDD
E6   NC   GVDD
E7   NC   GVDD
E8   NC   GVDD
E9   VSS   NC
E10   NC   GVDD
E11   VSS   NC
E12   NC   GVDD
E13   NC   BVDD
E14   VSS   NC
E15   NC   BVDD
E16   NC   BVDD
E17   NC   BVDD
E18   NC   BVDD
E19   NC   BVDD
E20   NC   BVDD
E21   NC   BVDD
E22   NC   BVDD
E23   NC   BVDD
E24   VSS   NC
E25   NC   BVDD
E26   NC   OVDD
E27   NC   OVDD
E28   NC   OVDD
E29   NC   OVDD
F1   NC   GVDD
F2   NC   GVDD
F3   NC   GVDD
F4   VSS   NC
F5   NC   GVDD
F6   NC   GVDD
F7   VSS   NC
F8   NC   GVDD
F9   NC   GVDD
F10   NC   GVDD
F11   NC   GVDD
F12   NC   GVDD
F13   VSS   NC
F14   NC   BVDD
F15   SENSEVSS   NC
F16   NC   BVDD
F17   NC   BVDD
F18   NC   BVDD
F19   NC   BVDD
F20   NC   BVDD
F21   NC   BVDD
F22   NC   BVDD
F23   NC   BVDD
F24   NC   OVDD
F25   NC   OVDD
F26   NC   OVDD
F27   NC   OVDD
F28   NC   OVDD
F29   NC   OVDD
G1   NC   GVDD
G2   NC   GVDD
G3   NC   GVDD
G4   NC   GVDD
G5   VSS   NC
G6   NC   GVDD
G9   NC   AVDD_CORE0
G10   VSS   NC
G20   NC   AVDD_CORE1
G21   VSS   NC
G24   NC   OVDD
G25   NC   OVDD
G26   NC   OVDD
G27   VSS   NC
G28   NC   OVDD
G29   NC   OVDD
H1   VSS   NC
H2   NC   GVDD
H3   NC   GVDD
H4   VSS   NC
H5   NC   GVDD
H6   NC   GVDD
H24   NC   OVDD
H25   NC   OVDD
H26   NC   OVDD
H27   NC   OVDD
H28   NC   OVDD
H29   VSS   NC
J1   NC   GVDD
J2   VSS   NC
J3   NC   GVDD
J4   NC   GVDD
J5   NC   GVDD
J6   NC   GVDD
J7   NC   GVDD
J23   NC   OVDD
J24   NC   OVDD
J25   NC   OVDD
J26   NC   OVDD
J27   NC   OVDD
J28   NC   OVDD
J29   NC   OVDD
K1   NC   GVDD
K2   NC   GVDD
K3   NC   GVDD
K4   NC   GVDD
K5   NC   GVDD
K6   VSS   NC
K7   VSS   NC
K10   NC   VDD
K11   NC   VDD
K12   NC   VDD
K13   NC   VDD
K14   NC   VDD
K15   NC   VDD
K16   NC   VDD
K17   NC   VDD
K18   NC   VDD
K19   NC   VDD
K20   NC   VDD
K23   VSS   NC
K24   NC   OVDD
K25   NC   OVDD
K26   NC   OVDD
K27   NC   OVDD
K28   NC   OVDD
K29   NC   OVDD
L1   NC   GVDD
L2   NC   GVDD
L3   VSS   NC
L4   NC   GVDD
L5   NC   GVDD
L6   NC   GVDD
L10   NC   VDD
L11   VSS   NC
L12   VSS   NC
L13   VSS   NC
L14   VSS   NC
L15   VSS   NC
L16   VSS   NC
L17   VSS   NC
L18   VSS   NC
L19   VSS   NC
L20   NC   VDD
L24   NC   OVDD
L25   NC   OVDD
L26   VSS   NC
L27   NC   O2VDD
L28   NC   OVDD
L29   NC   O2VDD
M1   VSS   NC
M2   NC   GVDD
M3   NC   GVDD
M4   VSS   NC
M5   NC   GVDD
M6   NC   GVDD
M10   NC   VDD
M11   VSS   NC
M12   VSS   NC
M13   VSS   NC
M14   VSS   NC
M15   VSS   NC
M16   VSS   NC
M17   VSS   NC
M18   VSS   NC
M19   VSS   NC
M20   NC   VDD
M24   NC   OVDD
M25   NC   O2VDD
M26   NC   O2VDD
M27   NC   O2VDD
M28   NC   O2VDD
M29   NC   OVDD
N1   NC   GVDD
N2   NC   GVDD
N3   NC   GVDD
N4   NC   GVDD
N5   NC   GVDD
N6   NC   GVDD
N10   NC   VDD
N11   VSS   NC
N12   VSS   NC
N13   VSS   NC
N14   VSS   NC
N15   VSS   NC
N16   VSS   NC
N17   VSS   NC
N18   VSS   NC
N19   VSS   NC
N20   NC   VDD
N24   NC   O2VDD
N25   NC   OVDD
N26   NC   O2VDD
N27   NC   OVDD
N28   NC   O2VDD
N29   VSS   NC
P1   NC   GVDD
P2   NC   GVDD
P3   NC   GVDD
P4   NC   GVDD
P5   VSS   NC
P6   NC   GVDD
P10   NC   VDDC
P11   VSS   NC
P12   VSS   NC
P13   VSS   NC
P14   VSS   NC
P15   VSS   NC
P16   VSS   NC
P17   VSS   NC
P18   VSS   NC
P19   VSS   NC
P20   NC   VDD
P24   NC   O2VDD
P25   NC   O2VDD
P26   NC   O2VDD
P27   NC   O2VDD
P28   NC   O2VDD
P29   NC   O2VDD
R1   NC   GVDD
R2   NC   GVDD
R3   NC   GVDD
R4   NC   GVDD
R5   NC   GVDD
R6   NC   GVDD
R10   NC   VDDC
R11   VSS   NC
R12   VSS   NC
R13   VSS   NC
R14   VSS   NC
R15   VSS   NC
R16   VSS   NC
R17   VSS   NC
R18   VSS   NC
R19   VSS   NC
R20   NC   VDD
R24   NC   O2VDD
R25   VSS   NC
R26   NC   O2VDD
R27   NC   O2VDD
R28   NC   O2VDD
R29   NC   O2VDD
T1   NC   GVDD
T2   NC   GVDD
T3   VSS   NC
T4   NC   GVDD
T5   NC   GVDD
T6   VSS   NC
T10   NC   VDD
T11   VSS   NC
T12   VSS   NC
T13   VSS   NC
T14   VSS   NC
T15   VSS   NC
T16   VSS   NC
T17   VSS   NC
T18   VSS   NC
T19   VSS   NC
T20   NC   VDD1C
T24   NC   O2VDD
T25   NC   O2VDD
T26   NC   O2VDD
T27   NC   O2VDD
T28   NC   O2VDD
T29   NC   O2VDD
U1   VSS   NC
U2   NC   GVDD
U3   NC   GVDD
U4   NC   GVDD
U5   NC   GVDD
U6   NC   GVDD
U10   NC   VDD
U11   VSS   NC
U12   VSS   NC
U13   VSS   NC
U14   VSS   NC
U15   VSS   NC
U16   VSS   NC
U17   VSS   NC
U18   VSS   NC
U19   VSS   NC
U20   NC   VDD1C
U24   NC   O2VDD
U25   VSS   NC
U26   NC   L2VDD
U27   NC   O2VDD
U28   NC   O2VDD
U29   NC   O2VDD
V1   NC   GVDD
V2   NC   GVDD
V3   VSS   NC
V4   NC   GVDD
V5   VSS   NC
V6   NC   GVDD
V10   NC   VDD
V11   VSS   NC
V12   VSS   NC
V13   VSS   NC
V14   VSS   NC
V15   VSS   NC
V16   VSS   NC
V17   VSS   NC
V18   VSS   NC
V19   VSS   NC
V20   NC   VDD
V24   NC   L2VDD
V25   NC   L2VDD
V26   NC   L2VDD
V27   NC   L2VDD
V28   NC   L2VDD
V29   NC   L2VDD
W1   NC   GVDD
W2   NC   GVDD
W3   NC   GVDD
W4   VSS   NC
W5   NC   GVDD
W6   VSS   NC
W10   NC   VDD
W11   VSS   NC
W12   VSS   NC
W16   VSS   NC
W18   VSS   NC
W19   VSS   NC
W20   NC   VDD
W24   NC   L2VDD
W25   VSS   NC
W26   NC   L2VDD
W27   NC   L2VDD
W28   NC   L2VDD
W29   VSS   NC
Y1   NC   GVDD
Y2   NC   GVDD
Y3   VSS   NC
Y4   NC   GVDD
Y5   NC   GVDD
Y6   NC   GVDD
Y7   NC   GVDD
Y10   NC   AVDD_DDR
Y11   NC   VDD
Y12   NC   VDD
Y16   NC   VDD
Y18   NC   VDD
Y19   NC   VDD
Y20   NC   VDD
Y23   VSS   NC
Y24   NC   L2VDD
Y25   NC   L2VDD
Y26   NC   L2VDD
Y27   NC   L2VDD
Y28   NC   L2VDD
Y29   NC   L2VDD
AA1   NC   GVDD
AA2   NC   GVDD
AA3   NC   GVDD
AA4   NC   GVDD
AA5   NC   GVDD
AA6   NC   GVDD
AA7   VSS   NC
AA23   NC   L2VDD
AA24   NC   L2VDD
AA25   NC   L2VDD
AA26   NC   L2VDD
AA27   NC   L2VDD
AA28   NC   L2VDD
AA29   VSS   NC
AB1   VSS   NC
AB2   NC   GVDD
AB3   NC   GVDD
AB4   NC   GVDD
AB5   NC   GVDD
AB6   NC   GVDD
AB24   NC   LVDD
AB25   NC   L2VDD
AB26   VSS   NC
AB27   NC   L2VDD
AB28   NC   L2VDD
AB29   NC   L2VDD
AC1   NC   GVDD
AC2   NC   GVDD
AC3   NC   GVDD
AC4   VSS   NC
AC5   NC   GVDD
AC6   NC   GVDD
AC20   NC   NC
AC21   X2VSS   NC
AC24   NC   LVDD
AC25   NC   LVDD
AC26   NC   LVDD
AC27   NC   LVDD
AC28   NC   LVDD
AC29   VSS   NC
AD1   NC   GVDD
AD2   NC   GVDD
AD3   NC   GVDD
AD4   NC   GVDD
AD5   NC   GVDD
AD6   VSS   NC
AD7   NC   O2VDD
AD8   XVSS   NC
AD9   NC   NC
AD10   NC   XVDD
AD11   NC   SDAVDD
AD12   SDAVSS   NC
AD13   NC   NC
AD14   NC   XVDD
AD15   NC   NC
AD16   XVSS   NC
AD17   X2VSS   NC
AD18   NC   NC
AD19   NC   SDAVDD2
AD20   X2VSS   NC
AD21   NC   NC
AD22   NC   X2VDD
AD23   VSS   NC
AD24   NC   LVDD
AD25   NC   LVDD
AD26   NC   LVDD
AD27   NC   LVDD
AD28   NC   LVDD
AD29   NC   L2VDD
AE1   VSS   NC
AE2   NC   GVDD
AE3   NC   GVDD
AE4   VSS   NC
AE5   NC   GVDD
AE6   NC   GVDD
AE7   VSS   NC
AE8   NC   XVDD
AE9   NC   NC
AE10   NC   NC
AE11   XVSS   NC
AE12   NC   NC
AE13   XVSS   NC
AE14   NC   NC
AE15   NC   NC
AE16   NC   XVDD
AE17   NC   NC
AE18   NC   X2VDD
AE19   SDAVSS2   NC
AE20   X2VSS   NC
AE21   NC   NC
AE22   NC   X2VDD
AE23   VSS   NC
AE24   NC   LVDD
AE25   NC   LVDD
AE26   NC   LVDD
AE27   VSS   NC
AE28   NC   LVDD
AE29   NC   LVDD
AF1   NC   GVDD
AF2   NC   GVDD
AF3   NC   GVDD
AF4   NC   GVDD
AF5   NC   GVDD
AF6   NC   GVDD
AF7   VSS   NC
AF8   XVSS   NC
AF9   XVSS   NC
AF10   NC   NC
AF11   NC   XVDD
AF12   NC   NC
AF13   NC   XVDD
AF14   NC   NC
AF15   XVSS   NC
AF16   NC   NC
AF17   NC   NC
AF18   S2VSS   NC
AF19   NC   NC
AF20   NC   X2VDD
AF21   S2VSS   NC
AF22   X2VSS   NC
AF24   VSS   NC
AF25   VSS   NC
AF26   NC   LVDD
AF27   NC   LVDD
AF28   VSS   NC
AF29   NC   LVDD
AG1   NC   GVDD
AG2   NC   GVDD
AG3   NC   GVDD
AG4   VSS   NC
AG5   NC   GVDD
AG6   NC   GVDD
AG7   VSS   NC
AG8   NC   NC
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| Diff Pairs
[Diff pin]   inv_pin   vdiff   tdelay_typ   tdelay_min   tdelay_max
|   MCK Signals
   H3   H2   250mV   0ns   NA   NA
   R3   R4   250mV   0ns   NA   NA
   K2   K3   250mV   0ns   NA   NA
   L2   L1   250mV   0ns   NA   NA
   N3   N4   250mV   0ns   NA   NA
   T4   T5   250mV   0ns   NA   NA
|   MDQS Signals: Use this format to arrange MDQS signals for
|   differential operation.  To use MDQS as
|   single-ended operation, comment out the following
|   nine lines.
   AG5   AH5   250mV   0ns   NA   NA
   AF1   AG1   250mV   0ns   NA   NA
   AB2   AB3   250mV   0ns   NA   NA
   AB5   AB4   250mV   0ns   NA   NA
   C2   C1   250mV   0ns   NA   NA
   B6   C6   250mV   0ns   NA   NA
   C9   D9   250mV   0ns   NA   NA
   B12   C12   250mV   0ns   NA   NA
   U2   U3   250mV   0ns   NA   NA
|   LYNX16 differential ports
|   SD_TX(0:3)
   AD9   AE9   NA   NA   NA   NA
   AE10   AF10   NA   NA   NA   NA
   AE14   AF14   NA   NA   NA   NA
   AD15   AE15   NA   NA   NA   NA
|   SD_RX(0:3)
   AH9   AJ9   NA   NA   NA   NA
   AH11   AJ11   NA   NA   NA   NA
   AH13   AJ13   NA   NA   NA   NA
   AH15   AJ15   NA   NA   NA   NA
|   SD_REF_CLK
   AG12   AF12   NA   NA   NA   NA
| LYNX18 differential ports
|   SD_TX(0:1)
   AE17   AF17   NA   NA   NA   NA
   AE21   AD21   NA   NA   NA   NA
|   SD_RX(0:1)
   AG18   AH18   NA   NA   NA   NA
   AH21   AG21   NA   NA   NA   NA
|   SD_REF_CLK
   AJ20   AJ19   NA   NA   NA   NA
|*   Model Selector   *
[Model Selector] ddr
ddr2_rcvr_150   DDR2 receiver with odt = 150 ohms
ddr2_rcvr_50   DDR2 receiver with odt =  50 ohms
ddr2_rcvr_75   DDR2 receiver with odt =  75 ohms
ddr2_rcvr_noterm   DDR2 receiver with no odt
ddr3_rcvr_120   DDR3 receiver with odt = 120 ohms
ddr3_rcvr_60   DDR3 receiver with odt = 60 ohms
ddr3_rcvr_noterm   DDR3 receiver with no odt
ddr2_drvr_18   DDR2 driver - 18 Ohm
ddr2_drvr_35   DDR2 driver - 35 Ohm
ddr3_drvr_17   DDR3 driver - 17 Ohm
ddr3_drvr_40   DDR23driver - 40 Ohm
[Model Selector] lvcmos
v180_in_wb   LVCMOS 1.8V Receiver
v250_in_wb   LVCMOS 2.5V Receiver
v330_in_wb   LVCMOS 3.3V Receiver
v180_wb   LVCMOS 1.8V IO
v250_wb   LVCMOS 2.5V IO
v330_wb   LVCMOS 3.3V IO
[Model Selector] lynx_tx
sd45_ohsdr100_x_004p serdes
sd45_ohsdr100_x_004s serdes
sd45_ohsdr100_x_006p serdes
sd45_ohsdr100_x_006s serdes
sd45_ohsdr100_x_303 serdes
sd45_ohsdr100_x_304 serdes
sd45_ohsdr100_x_403 serdes
sd45_ohsdr100_x_404 serdes
sd45_ohsdr100_x_502 serdes
sd45_ohsdr100_x_503 serdes
sd45_ohsdr100_x_602 serdes
sd45_ohsdr100_x_603 serdes
| Models and submodels in the file (49): ddr2_drvr_18 (I/O), ddr2_drvr_35 (I/O), ddr2_rcvr_150 (Input), ddr2_rcvr_50 (Input), ddr2_rcvr_75 (Input), ddr2_rcvr_noterm (Input), ddr3_drvr_17 (I/O), ddr3_drvr_40 (I/O), ddr3_rcvr_120 (Input), ddr3_rcvr_60 (Input), ddr3_rcvr_noterm (Input), opdalg_out (Output), pouv_out (3-state), v180_in_wb (Input), v330_in_wb (Input), v250_wb (I/O), v250_in_wb (Input), v180_wb (I/O), v330_wb (I/O), ptrmr100_cm (Input), rx_pzctl (Input), sd45_ohsdr100_x_004p (3-state), sd45_ohsdr100_x_004s (3-state), sd45_ohsdr100_x_006p (3-state), sd45_ohsdr100_x_006s (3-state), sd45_ohsdr100_x_304 (3-state), sd45_ohsdr100_x_303 (3-state), sd45_ohsdr100_x_403 (3-state), sd45_ohsdr100_x_502 (3-state), sd45_ohsdr100_x_503 (3-state), sd45_ohsdr100_x_602 (3-state), sd45_ohsdr100_x_603 (3-state), sd45_ohsdr100_x_00 (3-state), sd45_ohsdr100_x_04 (3-state), sd45_ohsdr100_x_06 (3-state), sd45_ohsdr100_x_30 (3-state), sd45_ohsdr100_x_33 (3-state), sd45_ohsdr100_x_34 (3-state), sd45_ohsdr100_x_40 (3-state), sd45_ohsdr100_x_43 (3-state), sd45_ohsdr100_x_44 (3-state), sd45_ohsdr100_x_50 (3-state), sd45_ohsdr100_x_52 (3-state), sd45_ohsdr100_x_53 (3-state), sd45_ohsdr100_x_60 (3-state), sd45_ohsdr100_x_62 (3-state), sd45_ohsdr100_x_63 (3-state), tx_pzctl (Input), sd45_ohsdr100_x_404 (3-state)
